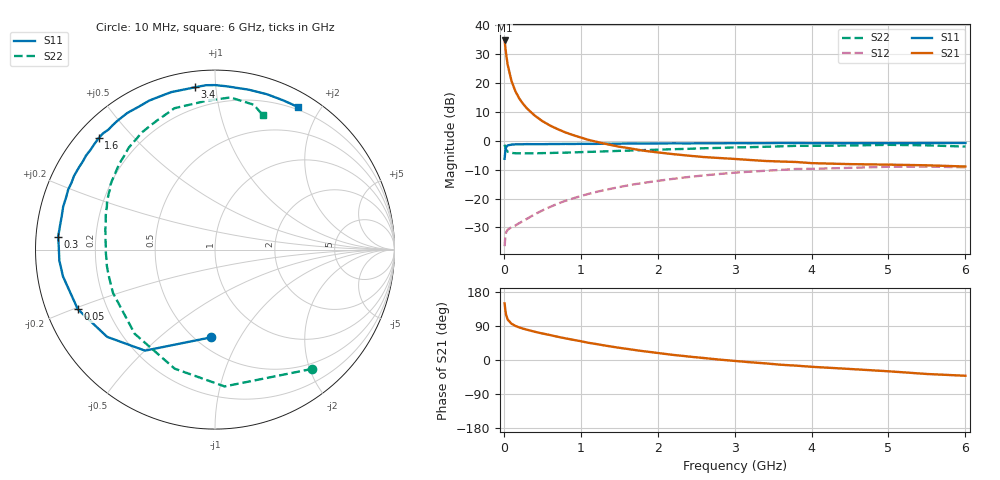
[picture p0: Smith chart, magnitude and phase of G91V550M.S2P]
! SIEMENS Small Signal Semiconductors
! BFG235
! Si NPN RF Bipolar Junction Transistor in SOT223
! VCE = 1.5 V  IC = 50 mA
! Common Emitter S-Parameters:  July  1994
# GHz  S  MA  R  50
!  f  S11  S21  S12  S22
! GHz  MAG  ANG  MAG  ANG  MAG  ANG  MAG  ANG
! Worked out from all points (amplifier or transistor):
!   40 points, 10 MHz to 6 GHz, reference 50 ohm
!   highest |S21| = 34.8 dB at 10 MHz (marker M1)
!   |S21| within 3 dB of that: start of sweep to 22.37 MHz
!   unconditionally stable (mu >= 1): 484 MHz to 1.561 GHz
!   at 200 MHz: K = 0.69, MSG = 21.6 dB, |S12| = -28.5 dB
!   at 1.5 GHz: K = 1.01, MAG = 6.3 dB, |S12| = -16.0 dB
!   at 6 GHz: K = 0.95, MSG = 0.1 dB, |S12| = -9.2 dB
!   S11 on the Smith chart (normalised r, x): 10 MHz: 0.59, -0.76; 50 MHz: 0.09, -0.21; 300 MHz: 0.07, +0.04; 1.6 GHz: 0.06, +0.40; 3.4 GHz: 0.08, +0.88; 6 GHz: 0.17, +1.73
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0.01  0.489 -92.4  54.68 149.5  0.015 61.0  0.8575 -50.8
0.02  0.6846 -124.7  41.21 130.1  0.0224 44.5  0.7642 -86.0
0.03  0.7729 -141.0  31.66 118.5  0.0261 35.6  0.7003 -108.7
0.05  0.8334 -156.5  20.68 106.8  0.0289 27.7  0.6481 -133.7
0.1  0.8601 -170.0  10.81 95.6  0.0321 27.5  0.6175 -157.0
0.15  0.8694 -176.0  7.24 89.9  0.0342 32.1  0.6098 -166.3
0.2  0.8695 -179.5  5.421 86.0  0.0376 36.1  0.6093 -171.5
0.25  0.8724 177.5  4.366 82.7  0.0409 40.2  0.6069 -175.0
0.3  0.8768 175.3  3.647 80.0  0.0446 43.8  0.6083 -177.8
0.4  0.8735 170.9  2.749 74.7  0.0534 48.4  0.6086 178.2
0.5  0.8744 167.3  2.199 70.0  0.0623 51.2  0.6124 175.0
0.6  0.8791 164.1  1.841 65.9  0.0716 52.5  0.6158 172.1
0.8  0.8837 157.8  1.399 57.2  0.0915 53.4  0.624 167.1
1.1  0.8857 148.8  1.04 45.4  0.1204 51.5  0.6436 160.5
1.3  0.8893 143.9  0.9 38.6  0.1397 49.2  0.6561 156.5
1.6  0.8976 136.2  0.756 29.4  0.1678 44.5  0.6745 150.1
2.2  0.9046 122.7  0.588 13.5  0.2198 34.2  0.7167 138.0
3.2  0.9085 101.3  0.466 -5.9  0.2925 15.1  0.7772 118.3
3.4  0.9109 97.1  0.448 -8.9  0.3031 11.1  0.7889 114.0
4.5  0.9106 78.1  0.395 -23.7  0.3405 -9.4  0.831 93.1
5.5  0.9144 65.3  0.377 -36.9  0.3582 -27.2  0.8355 75.0
6  0.9193 59.7  0.359 -41.6  0.3476 -33.9  0.7948 70.4
